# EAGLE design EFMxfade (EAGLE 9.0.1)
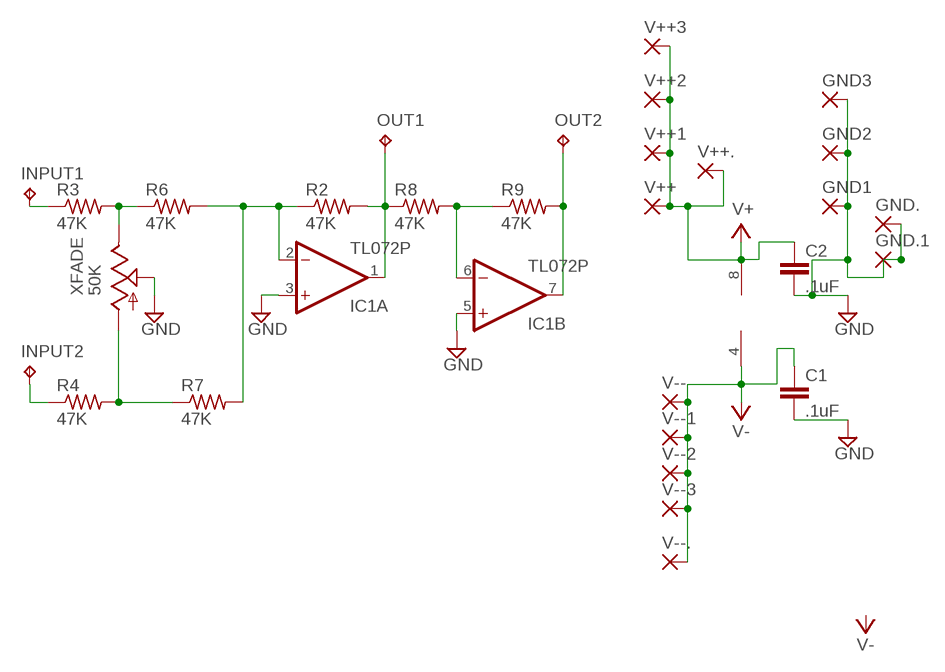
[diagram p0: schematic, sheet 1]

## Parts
C1  .1uF  C5/2.5  [C5B2.5]
C2  .1uF  C5/2.5  [C5B2.5]
GND1  3,17/1,1  [3,17/1,1]
GND2  3,17/1,1  [3,17/1,1]
GND3  3,17/1,1  [3,17/1,1]
GND.  1,6/0,9  [1,6/0,9]
GND.1  1,6/0,9  [1,6/0,9]
IC1  TL072P  [DIL08]
INPUT1  TPPAD1-17Y  [P1-17Y]
INPUT2  TPPAD1-17Y  [P1-17Y]
OUT1  TPPAD1-17Y  [P1-17Y]
OUT2  TPPAD1-17Y  [P1-17Y]
R2  47K  R-US_0204/7  [0204/7]
R3  47K  R-US_0204/7  [0204/7]
R4  47K  R-US_0204/7  [0204/7]
R6  47K  R-US_0204/7  [0204/7]
R7  47K  R-US_0204/7  [0204/7]
R8  47K  R-US_0204/7  [0204/7]
R9  47K  R-US_0204/7  [0204/7]
V++  3,17/1,1  [3,17/1,1]
V++1  3,17/1,1  [3,17/1,1]
V++2  3,17/1,1  [3,17/1,1]
V++3  3,17/1,1  [3,17/1,1]
V++.  1,6/0,9  [1,6/0,9]
V--  3,17/1,1  [3,17/1,1]
V--1  3,17/1,1  [3,17/1,1]
V--2  3,17/1,1  [3,17/1,1]
V--3  3,17/1,1  [3,17/1,1]
V--.  1,6/0,9  [1,6/0,9]
XFADE  50K  TRIM_US-S63X  [S63X]

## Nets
GND: C1.2 C2.2 GND1.1(P) GND2.1(P) GND3.1(P) GND.1.1(P) GND..1(P) IC1.3(A:+IN) IC1.5(B:+IN) XFADE.S
N$1: INPUT1.TP R3.1
N$2: R3.2 R6.1 XFADE.E
N$4: R4.2 R7.1 XFADE.A
N$5: INPUT2.TP R4.1
N$6: IC1.2(A:-IN) R2.1 R6.2 R7.2
N$7: IC1.1(A:OUT) OUT1.TP R2.2 R8.1
N$8: IC1.6(B:-IN) R8.2 R9.1
N$9: IC1.7(B:OUT) OUT2.TP R9.2
V+: C2.1 IC1.8(P:V+) V++1.1(P) V++2.1(P) V++3.1(P) V++.1(P) V++..1(P)
V-: C1.1 IC1.4(P:V-) V--1.1(P) V--2.1(P) V--3.1(P) V--.1(P) V--..1(P)

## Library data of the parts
C1 C2 = capacitor-wima:C: CAPACITOR
GND1-GND3 V++ V++1-V++3 V-- V--1-V--3 = wirepad-NONAMES:3,17/1,1: THROUGH-HOLE PAD
GND. GND.1 V++. V--. = wirepad-NONAMES:1,6/0,9: THROUGH-HOLE PAD
IC1 = linear:TL072: OP AMP
INPUT1 INPUT2 OUT1 OUT2 = testpad:TP: Test pad
R2-R4 R6-R9 = rcl:R-US_: RESISTOR, American symbol
XFADE = pot:TRIM_US-: POTENTIOMETER

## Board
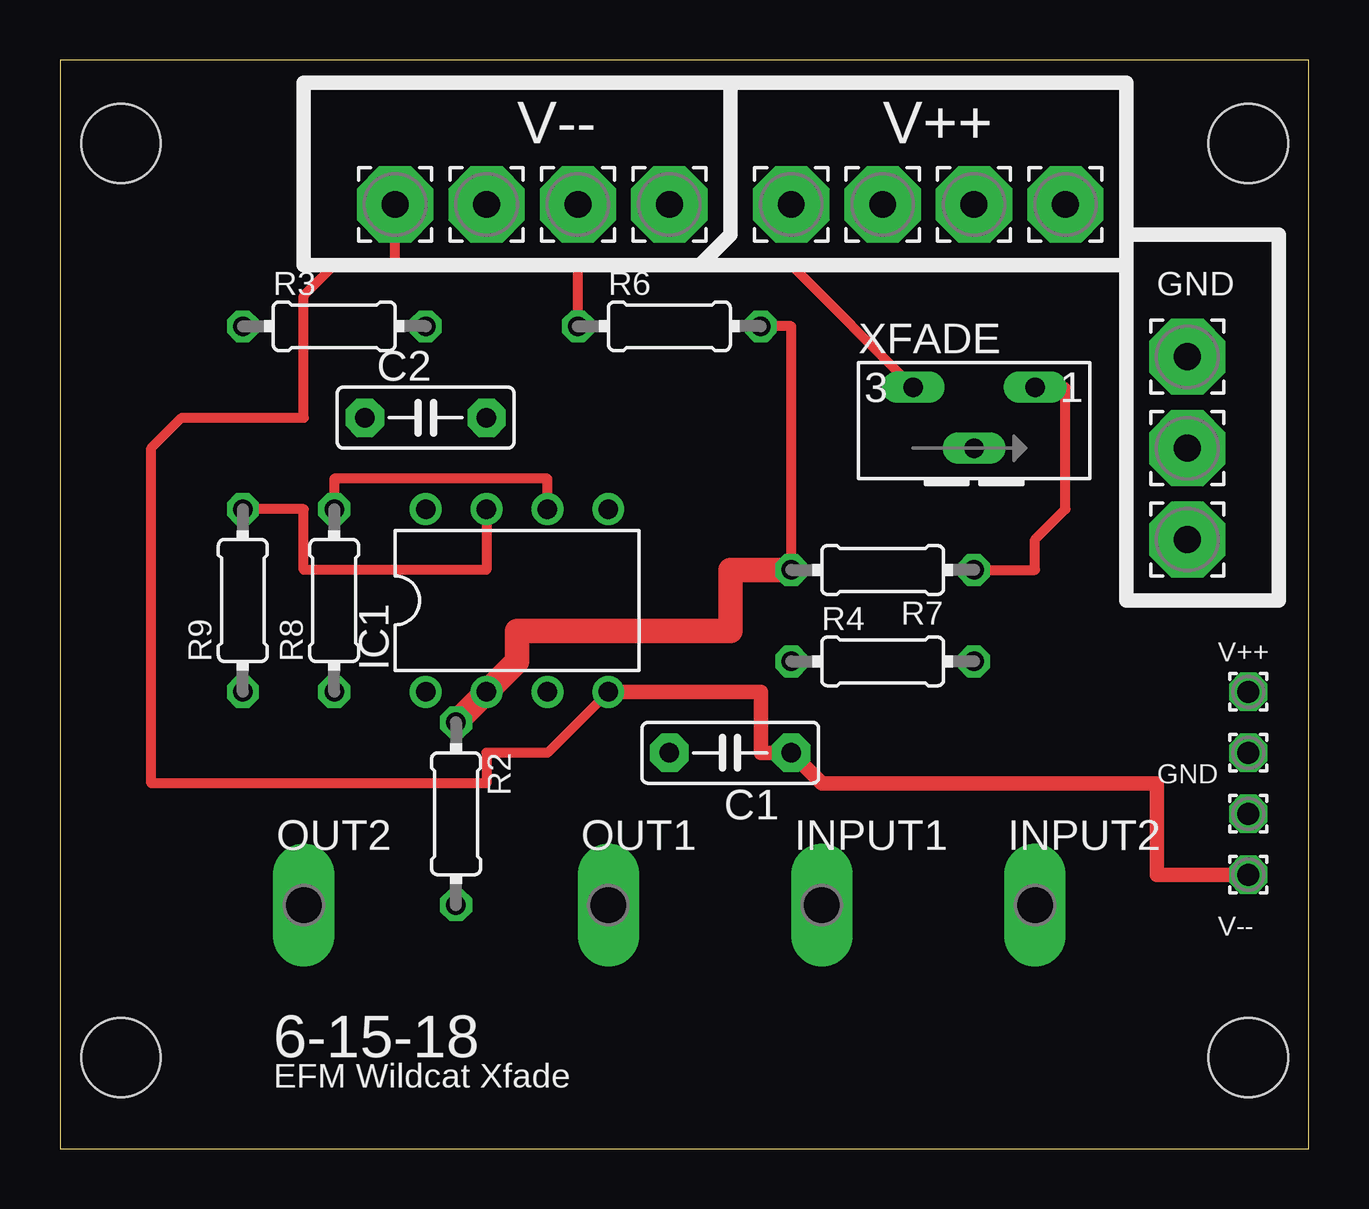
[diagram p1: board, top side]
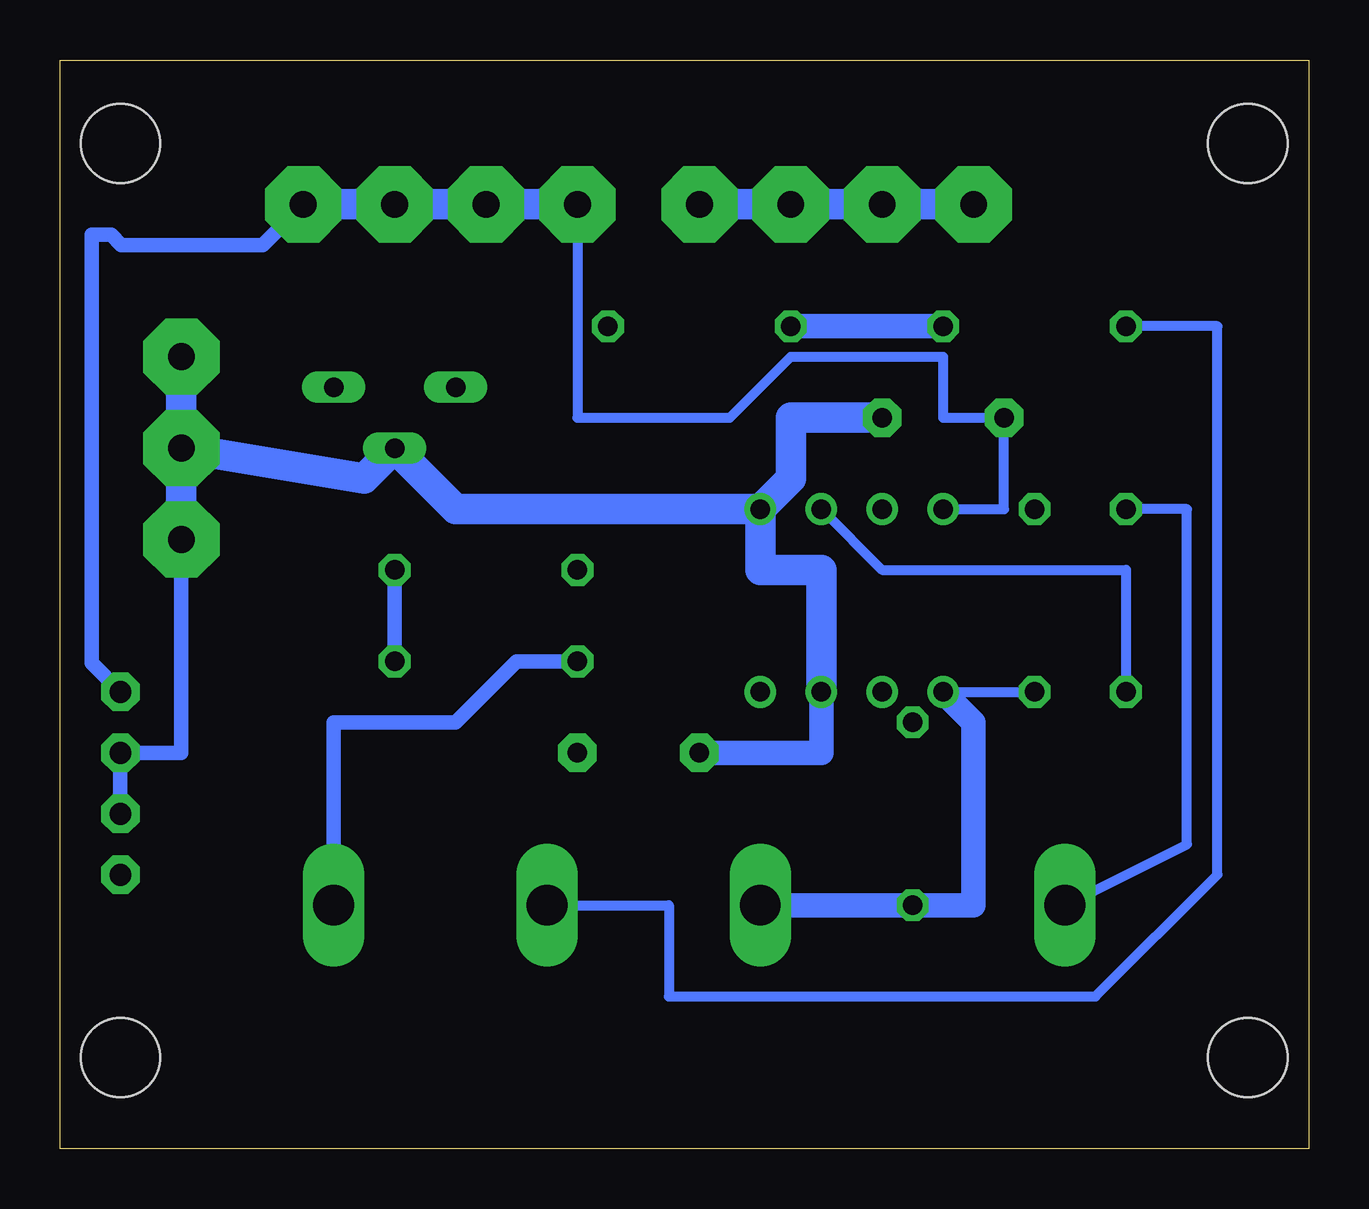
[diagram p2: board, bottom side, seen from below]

Size 52.05 x 45.39 mm. Coordinates in mm from the lower left corner, seen from the top.
Outline: 0,0 52.05,0 52.05,45.39 0,45.39 0,0
Copper layers (1*16): Top 0.035mm / dielectric 1.5mm / Bottom 0.035mm
Design rules "default": minimum track width 6mil, minimum drill 0.35mm, track to track 6mil, track to pad 6mil, pad to pad 6mil, via to via 6mil, smd to smd 6mil, copper to edge 40mil, drill to drill 6mil, minimum pad ring 10mil, minimum via ring 8mil, stop-mask expansion 4mil, vias tented up to drill 0mil, thermal gap 10mil
Holes 3.3 mm at 2.54,41.91 2.54,3.81 49.53,3.81 49.53,41.91

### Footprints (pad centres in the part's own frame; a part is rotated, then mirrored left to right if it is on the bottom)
C5B2.5 = drill 0.813 pad 1.6 octagon: 1 -2.54,0; 2 2.54,0
3,17/1,1 = drill 1.118 pad 3.175 octagon: 1 0,0
1,6/0,9 = drill 0.914 pad 1.6 octagon: 1 0,0
DIL08 = drill 0.813 pad 1.27: 1 -3.81,-3.81; 2 -1.27,-3.81; 3 1.27,-3.81; 4 3.81,-3.81; 5 3.81,3.81; 6 1.27,3.81; 7 -1.27,3.81; 8 -3.81,3.81
P1-17Y = drill 1.702 pad 2.121 long: TP 0,0
0204/7 = drill 0.813 octagon: 1 -3.81,0; 2 3.81,0
S63X = drill 0.813 long: A 2.54,0; E -2.54,0; S 0,-2.54

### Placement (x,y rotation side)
C1  27.94,16.51 180 top
C2  15.24,30.48 0 top
GND1  46.99,29.21 0 top
GND2  46.99,33.02 0 top
GND3  46.99,25.4 0 top
GND.  49.53,13.97 0 top
GND.1  49.53,16.51 0 top
IC1  19.05,22.86 0 top
INPUT1  31.75,10.16 0 top
INPUT2  40.64,10.16 0 top
OUT1  22.86,10.16 0 top
OUT2  10.16,10.16 0 top
R2  16.51,13.97 270 top
R3  11.43,34.29 0 top
R4  34.29,20.32 0 top
R6  25.4,34.29 0 top
R7  34.29,24.13 180 top
R8  11.43,22.86 90 top
R9  7.62,22.86 90 top
V++  34.29,39.37 0 top
V++1  41.91,39.37 0 top
V++2  30.48,39.37 0 top
V++3  38.1,39.37 0 top
V++.  49.53,19.05 0 top
V--  25.4,39.37 0 top
V--1  21.59,39.37 0 top
V--2  17.78,39.37 0 top
V--3  13.97,39.37 0 top
V--.  49.53,11.43 0 top
XFADE  38.1,31.75 0 top

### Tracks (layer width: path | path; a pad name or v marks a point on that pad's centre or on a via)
GND
  Bottom 0.61: GND..1 GND.1.1 46.99,16.51 GND3.1
  Bottom 1.016: C1.2 20.32,16.51 IC1.3
  Bottom 1.27: GND2.1 GND1.1 | GND1.1 GND3.1 | GND1.1 39.37,27.94 XFADE.S 35.56,26.67 IC1.5 | IC1.5 21.59,27.94 21.59,30.48 C2.2 | IC1.3 20.32,24.13 22.86,24.13 IC1.5
N$1
  Bottom 0.406: INPUT1.TP 26.67,10.16 26.67,6.35 8.89,6.35 3.81,11.43 3.81,34.29 R3.1
N$2
  Top 0.406: R6.1 21.59,36.83 30.48,36.83 XFADE.E
  Bottom 1.016: R3.2 R6.1
N$4
  Top 0.406: R7.1 40.64,24.13 40.64,25.4 41.91,26.67 41.91,31.75 XFADE.A
  Bottom 0.61: R4.2 R7.1
N$5
  Bottom 0.61: R4.1 33.02,20.32 35.56,17.78 40.64,17.78 INPUT2.TP
N$6
  Top 0.406: R7.2 30.48,34.29 R6.2
  Top 1.016: R2.1 IC1.2 19.05,20.32 19.05,21.59 27.94,21.59 27.94,24.13 R7.2
N$7
  Bottom 0.406: IC1.1 R8.1
  Bottom 1.016: OUT1.TP R2.2 13.97,10.16 13.97,17.78 IC1.1
N$8
  Top 0.406: IC1.6 20.32,27.94 11.43,27.94 R8.2
  Bottom 0.406: IC1.6 17.78,24.13 7.62,24.13 R9.1
N$9
  Top 0.406: IC1.7 17.78,24.13 10.16,24.13 10.16,26.67 R9.2
  Bottom 0.406: OUT2.TP 5.08,12.7 5.08,26.67 R9.2
V+
  Bottom 0.406: IC1.8 12.7,26.67 C2.1 15.24,30.48 15.24,33.02 21.59,33.02 24.13,30.48 30.48,30.48 V++2.1
  Bottom 0.61: V++..1 50.73,20.25 50.73,38.1 49.92,38.1 49.49,37.67 43.61,37.67 V++1.1
  Bottom 1.27: V++2.1 V++.1 V++3.1 V++1.1
V-
  Top 0.406: IC1.4 20.32,16.51 17.78,16.51 17.78,15.24 3.81,15.24 3.81,29.21 5.08,30.48 10.16,30.48 10.16,35.56 11.43,36.83 13.97,36.83 V--3.1
  Top 0.61: IC1.4 29.21,19.05 29.21,16.51 C1.1 31.75,15.24 45.72,15.24 45.72,11.43 V--..1
  Bottom 1.27: V--3.1 V--2.1 V--1.1 V--.1

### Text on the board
tNames: V-- | V++ | GND | V++ | GND | V-- | 6-15-18 | EFM Wildcat Xfade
